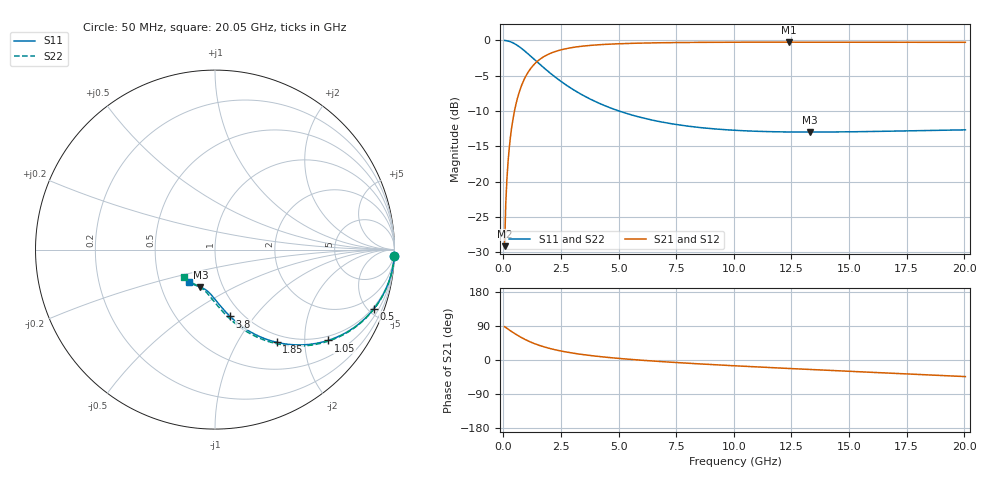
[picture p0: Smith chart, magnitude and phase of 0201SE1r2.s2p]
! AVX Thin Film Operation		Date: August 2001
! Description: Accu-P® Series, Thin Film, SMD, RF Capacitor
! Part Number: 02013J1R2ABW
! 50 MHz  -  20.05 GHz
! Serial Measurements
# mhz S db R 50
!	S11		S21		S12		S22
!	dB	Phase	dB	Phase	dB	Phase	dB	Phase
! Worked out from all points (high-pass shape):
!   401 points, 50 MHz to 20.05 GHz, reference 50 ohm
!   highest |S21| = -0.24 dB at 12.4 GHz (marker M1); lowest = -29.1 dB at 50 MHz (marker M2)
!   |S21| within 3 dB of the highest: 1.378 GHz to end of sweep
!   lowest |S11| = -13.0 dB at 13.3 GHz (marker M3), VSWR 1.58, Z = 39.1 - j17.2 ohm
!   |S11| at or under -10 dB: 5.019 GHz to end of sweep
!   |S22| runs from -13.0 to 0.0 dB; largest |S21 - S12| = 0
!   S11 on the Smith chart (normalised r, x): 50 MHz: 1, -54; 500 MHz: 0.88, -5.39; 1.05 GHz: 0.88, -2.58; 1.85 GHz: 0.88, -1.48; 3.8 GHz: 0.87, -0.76; 20.05 GHz: 0.70, -0.27
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50  -0.01 -2.1  -29.14 87.9  -29.14 87.9  -0.01 -2.2
100  -0.02 -4.3  -23.14 85.7  -23.14 85.7  -0.02 -4.3
200  -0.08 -8.5  -17.18 81.5  -17.18 81.5  -0.08 -8.6
250  -0.13 -10.5  -15.29 79.4  -15.29 79.4  -0.13 -10.7
350  -0.25 -14.6  -12.49 75.3  -12.49 75.3  -0.25 -14.8
500  -0.50 -20.5  -9.65 69.3  -9.65 69.3  -0.50 -20.8
750  -1.05 -29.5  -6.70 60.3  -6.70 60.3  -1.05 -29.9
1050  -1.85 -38.8  -4.61 50.9  -4.61 50.9  -1.85 -39.3
1400  -2.86 -47.6  -3.17 42.0  -3.17 42.0  -2.86 -48.3
1850  -4.15 -56.4  -2.12 33.1  -2.12 33.1  -4.15 -57.4
2200  -5.08 -61.7  -1.63 27.6  -1.63 27.6  -5.08 -62.9
2550  -5.93 -66.2  -1.29 23.1  -1.29 23.1  -5.93 -67.5
3400  -7.68 -74.3  -0.82 14.7  -0.82 14.7  -7.68 -76.1
3800  -8.36 -77.2  -0.70 11.6  -0.70 11.6  -8.37 -79.2
5050  -10.04 -84.5  -0.47 4.0  -0.47 4.0  -10.04 -87.1
6750  -11.48 -91.8  -0.33 -3.8  -0.33 -3.8  -11.49 -95.2
10050  -12.73 -102.4  -0.25 -15.3  -0.25 -15.3  -12.76 -107.3
12400  -12.97 -108.9  -0.24 -22.4  -0.24 -22.4  -13.00 -114.8
13300  -12.98 -111.3  -0.24 -25.0  -0.24 -25.0  -13.02 -117.6
13400  -12.98 -111.5  -0.24 -25.3  -0.24 -25.3  -13.02 -117.9
16750  -12.86 -120.2  -0.26 -34.7  -0.26 -34.7  -12.91 -128.0
20050  -12.67 -128.5  -0.27 -43.8  -0.27 -43.8  -12.73 -137.8
